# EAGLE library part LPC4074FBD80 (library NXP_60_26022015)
32-bit ARM Cortex-M4 MCU; up to 512 kB flash, 96 kB SRAM; USB Device/Host/OTG; Ethernet; LCD; EMC; SPIFI The LPC408x/7x is an ARM Cortex-M4 based digital signal controller for embedded applications requiring a high level of integration and low power dissipation. The ARM Cortex-M4 is a next generation core that offers system enhancements such as low power consumption, enhanced debug features, and a high level of support block integration. The ARM Cortex-M4 CPU incorporates a 3-stage pipeline, uses a Harvard architecture with separate local instruction and data buses as well as a third bus for peripherals, and includes an internal prefetch unit that supports speculative branching. The ARM Cortex-M4 supports single-cycle digital signal processing and SIMD instructions. A hardware floating-point processor is integrated in the core for several versions of the part. The LPC408x/7x adds a specialized flash memory accelerator to accomplish optimal performance when executing code from flash. The LPC408x/7x is targeted to operate at up to 120 MHz CPU frequency. The peripheral complement of the LPC408x/7x includes up to 512 kB of flash program memory, up to 96 kB of SRAM data memory, up to 4032 byte of EEPROM data memory, External Memory controller (EMC), LCD, Ethernet, USB Device/Host/OTG, an SPI Flash Interface (SPIFI), a General Purpose DMA controller, five UARTs, three SSP controllers, three I 2 C-bus interfaces, a Quadrature Encoder Interface, four general purpose timers, two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
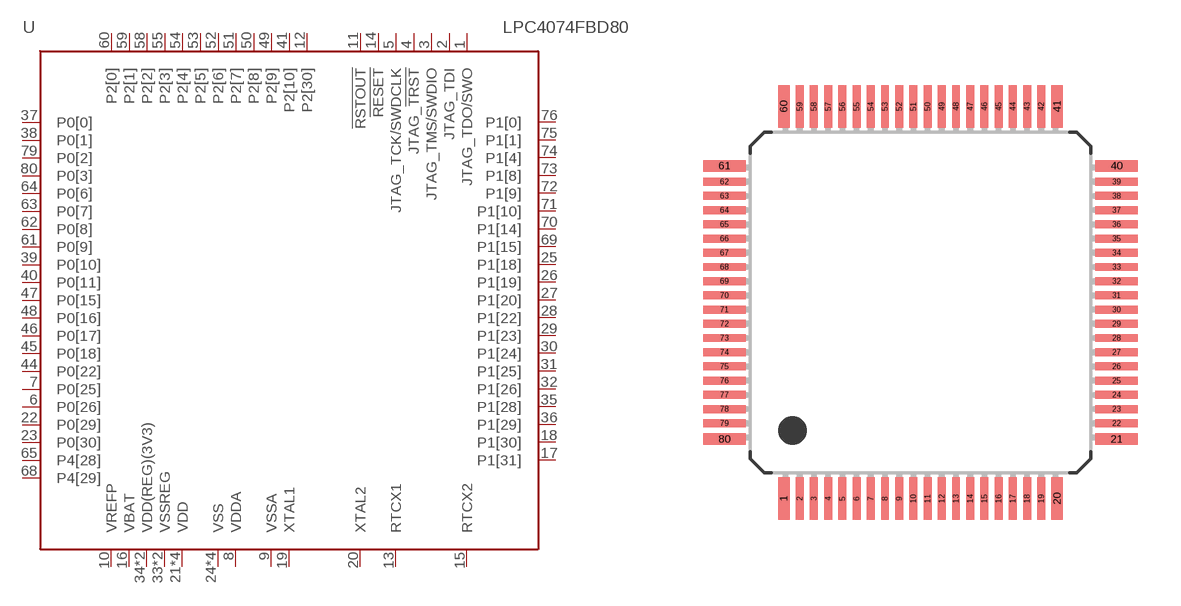
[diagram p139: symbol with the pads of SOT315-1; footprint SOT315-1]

Designator prefix U

## LPC4074FBD80  [SOT315-1]
1  JTAG_TDO/SWO  out
2  JTAG_TDI  in
3  JTAG_TMS/SWDIO  in
4  JTAG_!TRST  in
5  JTAG_TCK/SWDCLK  in
6  P0[26]
7  P0[25]
8  VDDA  pwr
9  VSSA  pwr
10  VREFP  pwr
11  !RSTOUT!  out
12  P2[30]
13  RTCX1  in
14  !RESET!  in
15  RTCX2  out
16  VBAT  pwr
17  P1[31]
18  P1[30]
19  XTAL1  in
20  XTAL2  out
21  VDD  pwr
22  P0[29]
23  P0[30]
24  VSS  pwr
25  P1[18]
26  P1[19]
27  P1[20]
28  P1[22]
29  P1[23]
30  P1[24]
31  P1[25]
32  P1[26]
33  VSSREG  pwr
34  VDD(REG)(3V3)  pwr
35  P1[28]
36  P1[29]
37  P0[0]
38  P0[1]
39  P0[10]
40  P0[11]
41  P2[10]
42  VDD  pwr
43  VSS  pwr
44  P0[22]
45  P0[18]
46  P0[17]
47  P0[15]
48  P0[16]
49  P2[9]
50  P2[8]
51  P2[7]
52  P2[6]
53  P2[5]
54  P2[4]
55  P2[3]
56  VDD  pwr
57  VSS  pwr
58  P2[2]
59  P2[1]
60  P2[0]
61  P0[9]
62  P0[8]
63  P0[7]
64  P0[6]
65  P4[28]
66  VSSREG  pwr
67  VDD(REG)(3V3)  pwr
68  P4[29]
69  P1[15]
70  P1[14]
71  P1[10]
72  P1[9]
73  P1[8]
74  P1[4]
75  P1[1]
76  P1[0]
77  VDD  pwr
78  VSS  pwr
79  P0[2]
80  P0[3]

## Footprint SOT315-1 (pad centres in mm)
SOT315-1 LQFP80: plastic low profile quad flat package; 80 leads; body 12 x 12 x 1.4 mm JEDEC: MS-026 IEC: 136E15
smd 0.4 x 1.5: 1 -4.81,-6.9; 20 4.81,-6.9; 41 4.81,6.9; 60 -4.81,6.9
smd 0.28 x 1.5: 2 -4.25,-6.9; 3 -3.75,-6.9; 4 -3.25,-6.9; 5 -2.75,-6.9; 6 -2.25,-6.9; 7 -1.75,-6.9; 8 -1.25,-6.9; 9 -0.75,-6.9; 10 -0.25,-6.9; 11 0.25,-6.9; 12 0.75,-6.9; 13 1.25,-6.9; 14 1.75,-6.9; 15 2.25,-6.9; 16 2.75,-6.9; 17 3.25,-6.9; 18 3.75,-6.9; 19 4.25,-6.9; 42 4.25,6.9; 43 3.75,6.9; 44 3.25,6.9; 45 2.75,6.9; 46 2.25,6.9; 47 1.75,6.9; 48 1.25,6.9; 49 0.75,6.9; 50 0.25,6.9; 51 -0.25,6.9; 52 -0.75,6.9; 53 -1.25,6.9; 54 -1.75,6.9; 55 -2.25,6.9; 56 -2.75,6.9; 57 -3.25,6.9; 58 -3.75,6.9; 59 -4.25,6.9
smd 1.5 x 0.4: 21 6.9,-4.81; 40 6.9,4.81; 61 -6.9,4.81; 80 -6.9,-4.81
smd 1.5 x 0.28: 22 6.9,-4.25; 23 6.9,-3.75; 24 6.9,-3.25; 25 6.9,-2.75; 26 6.9,-2.25; 27 6.9,-1.75; 28 6.9,-1.25; 29 6.9,-0.75; 30 6.9,-0.25; 31 6.9,0.25; 32 6.9,0.75; 33 6.9,1.25; 34 6.9,1.75; 35 6.9,2.25; 36 6.9,2.75; 37 6.9,3.25; 38 6.9,3.75; 39 6.9,4.25; 62 -6.9,4.25; 63 -6.9,3.75; 64 -6.9,3.25; 65 -6.9,2.75; 66 -6.9,2.25; 67 -6.9,1.75; 68 -6.9,1.25; 69 -6.9,0.75; 70 -6.9,0.25; 71 -6.9,-0.25; 72 -6.9,-0.75; 73 -6.9,-1.25; 74 -6.9,-1.75; 75 -6.9,-2.25; 76 -6.9,-2.75; 77 -6.9,-3.25; 78 -6.9,-3.75; 79 -6.9,-4.25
